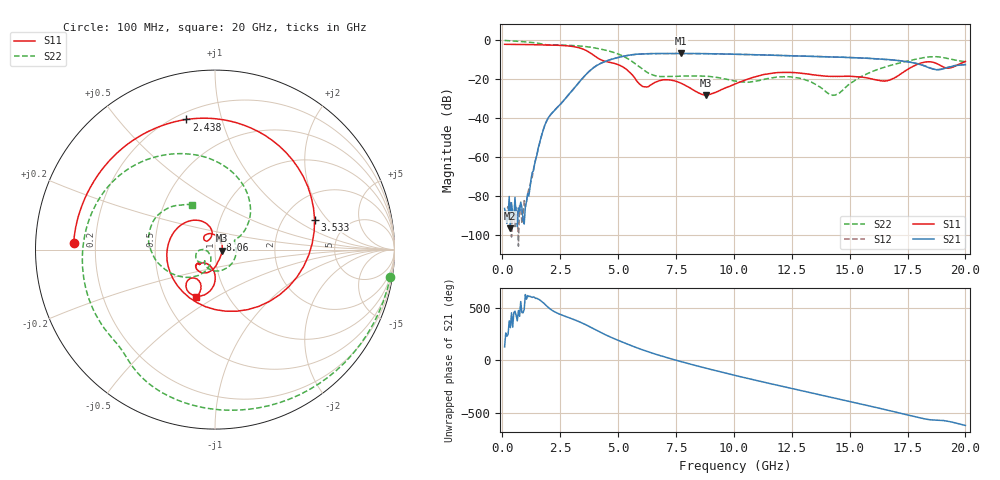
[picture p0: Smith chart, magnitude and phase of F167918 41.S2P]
!  2-Port S-parameters saved by WinCal
! VAR MeasName=S-Parameters (CALIBRATED_DATA) read from VNA (N5242A)
! VAR MeasDate=2016-11-22 10:26:44
! VAR NAME=F167918 41
! VAR FILENAME=F167918 41.S2P
! VAR DATE=2016-11-22 10:26:44
! VAR PHYS_PORTS=1,2
# Hz S DB R 50
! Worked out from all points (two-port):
!   401 points, 100 MHz to 20 GHz, reference 50 ohm
!   highest |S21| = -6.78 dB at 7.712 GHz (marker M1); lowest = -96.4 dB at 348.8 MHz (marker M2)
!   |S21| within 3 dB of the highest: 4.711 GHz to 16.47 GHz (11.76 GHz wide, 111 % of centre)
!   lowest |S11| = -28.1 dB at 8.806 GHz (marker M3), VSWR 1.08, Z = 54 - j0.633 ohm
!   |S11| at or under -10 dB: 4.259 GHz to end of sweep
!   |S22| runs from -28.2 to -0.1 dB; largest |S21 - S12| = 0.0052
!   S11 on the Smith chart (normalised r, x): 100 MHz: 0.12, +0.02; 2.438 GHz: 0.24, +0.78; 3.533 GHz: 2.94, +1.48; 8.06 GHz: 1.05, +0.12; 20 GHz: 0.71, -0.41
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1e8  -2.07 177.3  -86.20 127.6  -89.69 -45.4  -0.10 -8.8
3.4875e8  -2.09 170.7  -96.43 -49.9  -83.22 124.9  -0.26 -29.1
1.095e9  -2.22 150.4  -78.64 -105.4  -79.10 -133.1  -0.92 -84.6
1.7915e9  -2.36 128.6  -45.01 -177.9  -45.02 -178.5  -2.09 -127.6
2.43825e9  -2.59 102.4  -33.66 81.4  -33.69 81.0  -2.44 -156.0
3.43325e9  -4.28 28.7  -19.90 -4.7  -19.92 -4.5  -3.02 157.0
3.53275e9  -4.74 16.7  -18.57 -14.8  -18.59 -14.7  -3.14 152.1
4.03025e9  -8.39 -61.5  -13.31 -71.0  -13.27 -70.8  -4.01 127.6
4.5775e9  -11.15 -160.0  -10.30 -130.3  -10.25 -130.6  -5.43 100.5
5.42325e9  -15.54 112.5  -7.75 151.7  -7.76 151.4  -9.47 55.4
6.11975e9  -23.84 119.4  -6.95 94.3  -6.95 94.1  -15.30 29.8
6.7665e9  -20.77 133.4  -6.81 47.5  -6.82 47.4  -18.53 23.6
7.71175e9  -21.97 88.0  -6.78 -12.4  -6.81 -12.5  -18.40 -18.5
8.06e9  -24.11 65.0  -6.80 -33.2  -6.81 -33.3  -18.32 -41.0
8.80625e9  -28.13 -8.6  -6.88 -76.2  -6.88 -76.3  -18.42 -87.1
1.005e10  -22.40 -79.8  -7.14 -143.9  -7.15 -143.8  -20.92 -130.8
1.19405e10  -16.53 -121.7  -7.80 119.7  -7.76 119.6  -18.77 -145.4
1.338325e10  -17.66 -141.7  -8.26 48.7  -8.21 48.8  -21.66 -178.9
1.437825e10  -18.54 -137.9  -8.61 -0.0  -8.56 -0.1  -28.10 -139.5
1.67165e10  -20.50 -106.1  -9.92 -118.3  -9.97 -118.2  -13.06 -135.9
1.815925e10  -11.38 -106.8  -12.85 166.3  -12.74 166.4  -9.00 -178.4
2e10  -10.84 -111.7  -12.54 100.5  -12.42 100.3  -11.02 117.1
